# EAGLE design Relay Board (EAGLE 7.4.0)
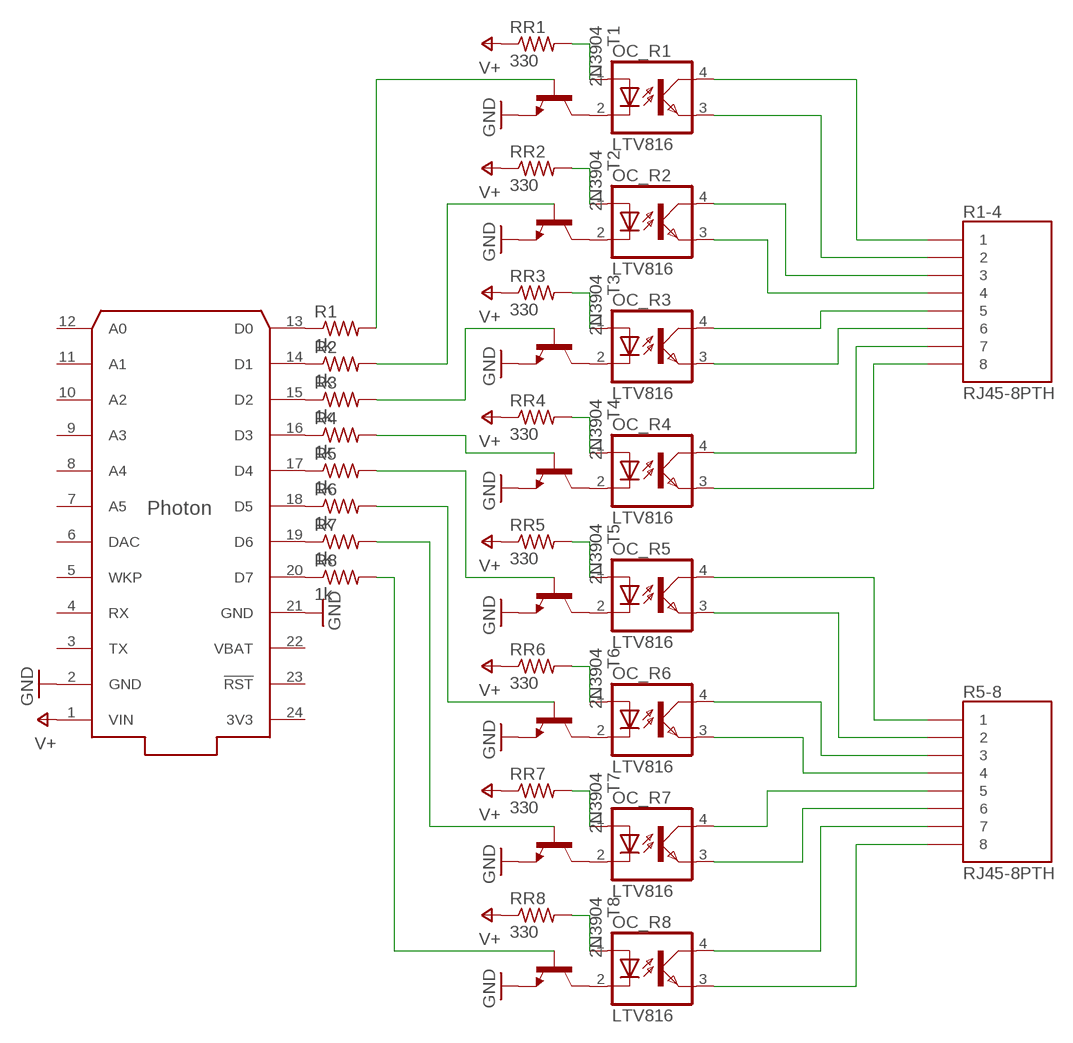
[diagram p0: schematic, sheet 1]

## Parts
OC_R1  LTV816  [DIL04]
OC_R2  LTV816  [DIL04]
OC_R3  LTV816  [DIL04]
OC_R4  LTV816  [DIL04]
OC_R5  LTV816  [DIL04]
OC_R6  LTV816  [DIL04]
OC_R7  LTV816  [DIL04]
OC_R8  LTV816  [DIL04]
PHOTON  PHOTON_WITH_HEADERS  [PHOTON]
R1  1k  R-US_0204/7  [0204/7]
R1-4  RJ45-8PTH  [RJ45-8]
R2  1k  R-US_0204/7  [0204/7]
R3  1k  R-US_0204/7  [0204/7]
R4  1k  R-US_0204/7  [0204/7]
R5  1k  R-US_0204/7  [0204/7]
R5-8  RJ45-8PTH  [RJ45-8]
R6  1k  R-US_0204/7  [0204/7]
R7  1k  R-US_0204/7  [0204/7]
R8  1k  R-US_0204/7  [0204/7]
RR1  330  R-US_0204/7  [0204/7]
RR2  330  R-US_0204/7  [0204/7]
RR3  330  R-US_0204/7  [0204/7]
RR4  330  R-US_0204/7  [0204/7]
RR5  330  R-US_0204/7  [0204/7]
RR6  330  R-US_0204/7  [0204/7]
RR7  330  R-US_0204/7  [0204/7]
RR8  330  R-US_0204/7  [0204/7]
T1  2N3904  [TO92]
T2  2N3904  [TO92]
T3  2N3904  [TO92]
T4  2N3904  [TO92]
T5  2N3904  [TO92]
T6  2N3904  [TO92]
T7  2N3904  [TO92]
T8  2N3904  [TO92]

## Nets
GND: PHOTON.2(GND) PHOTON.21(GND) T1.3(E) T2.3(E) T3.3(E) T4.3(E) T5.3(E) T6.3(E) T7.3(E) T8.3(E)
N$1: PHOTON.13(D0) R1.1
N$2: PHOTON.14(D1) R2.1
N$3: PHOTON.15(D2) R3.1
N$4: PHOTON.16(D3) R4.1
N$5: PHOTON.17(D4) R5.1
N$6: PHOTON.18(D5) R6.1
N$7: PHOTON.19(D6) R7.1
N$8: PHOTON.20(D7) R8.1
N$9: OC_R1.4(COL) R1-4.1
N$10: OC_R1.3(EMIT) R1-4.2
N$11: OC_R2.4(COL) R1-4.3
N$12: OC_R2.3(EMIT) R1-4.4
N$13: OC_R3.4(COL) R1-4.5
N$14: OC_R3.3(EMIT) R1-4.6
N$15: OC_R4.4(COL) R1-4.7
N$16: OC_R4.3(EMIT) R1-4.8
N$17: OC_R5.4(COL) R5-8.1
N$18: OC_R5.3(EMIT) R5-8.2
N$19: OC_R6.4(COL) R5-8.3
N$20: OC_R6.3(EMIT) R5-8.4
N$21: OC_R7.4(COL) R5-8.5
N$22: OC_R7.3(EMIT) R5-8.6
N$23: OC_R8.4(COL) R5-8.7
N$24: OC_R8.3(EMIT) R5-8.8
N$25: OC_R8.2(C) T8.1(C)
N$26: OC_R7.2(C) T7.1(C)
N$27: OC_R6.2(C) T6.1(C)
N$28: OC_R5.2(C) T5.1(C)
N$29: OC_R4.2(C) T4.1(C)
N$30: OC_R3.2(C) T3.1(C)
N$31: OC_R2.2(C) T2.1(C)
N$32: OC_R1.2(C) T1.1(C)
N$33: OC_R1.1(A) RR1.2
N$34: OC_R2.1(A) RR2.2
N$35: OC_R3.1(A) RR3.2
N$36: OC_R4.1(A) RR4.2
N$37: OC_R5.1(A) RR5.2
N$38: OC_R6.1(A) RR6.2
N$39: OC_R7.1(A) RR7.2
N$40: OC_R8.1(A) RR8.2
N$41: R1.2 T1.2(B)
N$42: R2.2 T2.2(B)
N$43: R3.2 T3.2(B)
N$44: R4.2 T4.2(B)
N$45: R5.2 T5.2(B)
N$46: R6.2 T6.2(B)
N$47: R7.2 T7.2(B)
N$48: R8.2 T8.2(B)
V+: PHOTON.1(VIN) RR1.1 RR2.1 RR3.1 RR4.1 RR5.1 RR6.1 RR7.1 RR8.1
Unconnected: PHOTON.3(TX) PHOTON.4(RX) PHOTON.5(WKP) PHOTON.6(DAC) PHOTON.7(A5) PHOTON.8(A4) PHOTON.9(A3) PHOTON.10(A2) PHOTON.11(A1) PHOTON.12(A0) PHOTON.23(!RST)

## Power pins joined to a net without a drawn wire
3V3: PHOTON.24(3V3)
VBAT: PHOTON.22(VBAT)

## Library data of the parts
OC_R1-OC_R8 = optocoupler:LTV816: OPTO COUPLER Source: LITEON, LTV816.pdf; OC_FARNELL: unknown; OC_NEWARK: unknown
PHOTON = Spark:PHOTON
R1-R8 RR1-RR8 = rcl:R-US_: RESISTOR, American symbol
R1-4 R5-8 = SparkFun-Connectors:RJ45-8: RJ45 Jack Simple RJ45, 8-pin connection - connector for common Cat5, Cat5e, and Cat6 Ethernet cables. Footprint not yet proven in production. Connector sku is PRT-00643; Breakout PCB sku is BOB-00716.
T1-T8 = transistor:2N3904: NPN TRANSISTOR

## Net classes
0 default: width 0.305 mm, drill 0.508 mm, clearance 0.254 mm

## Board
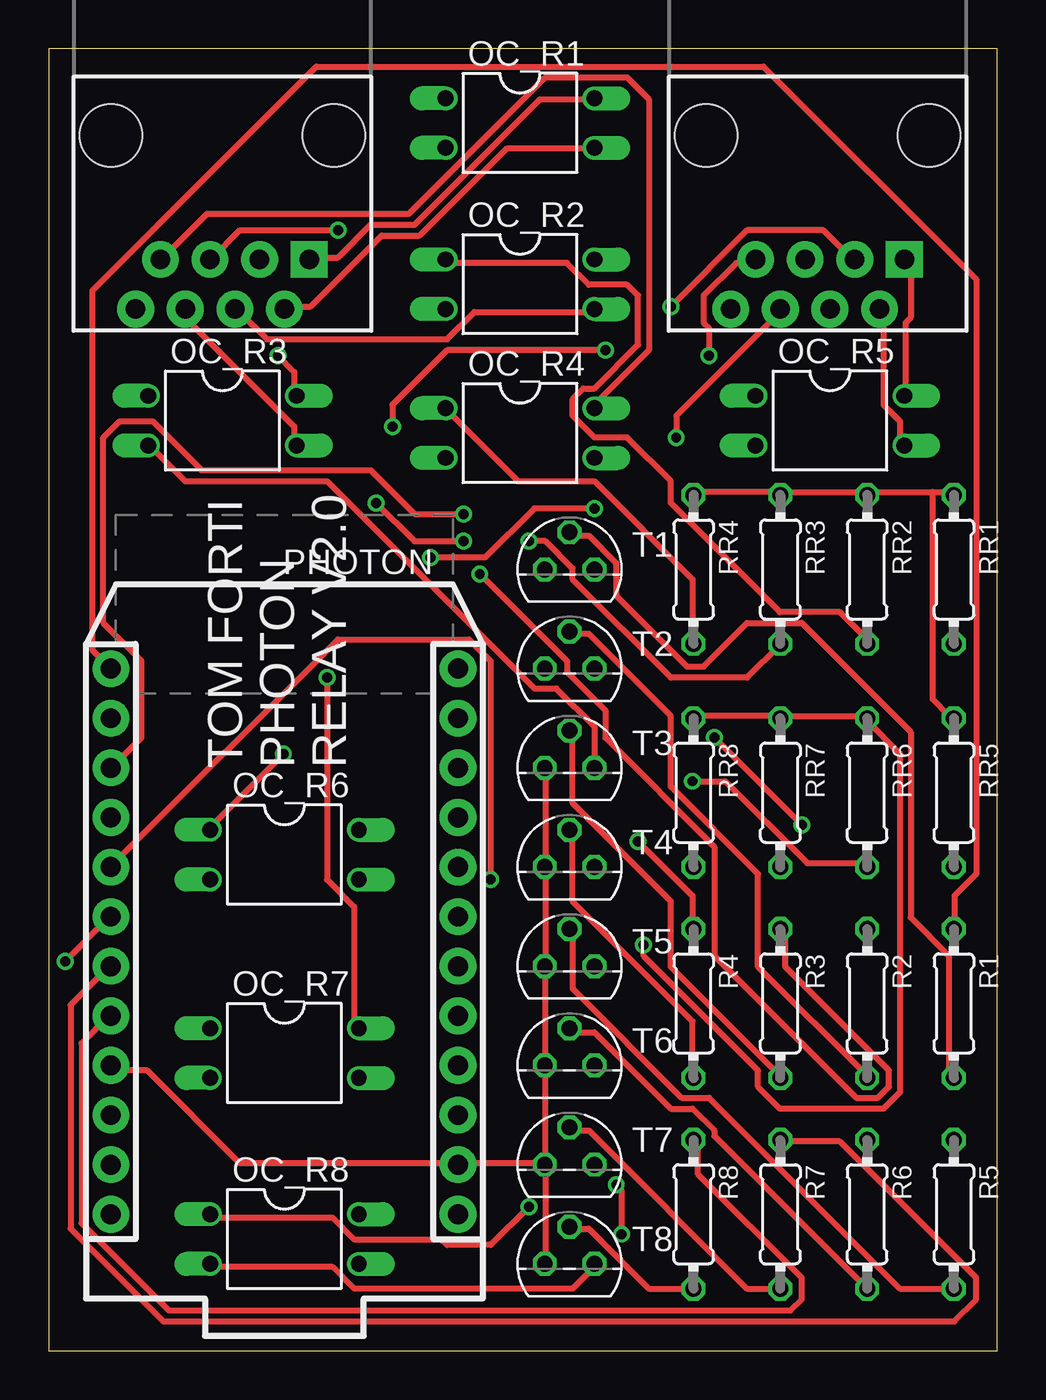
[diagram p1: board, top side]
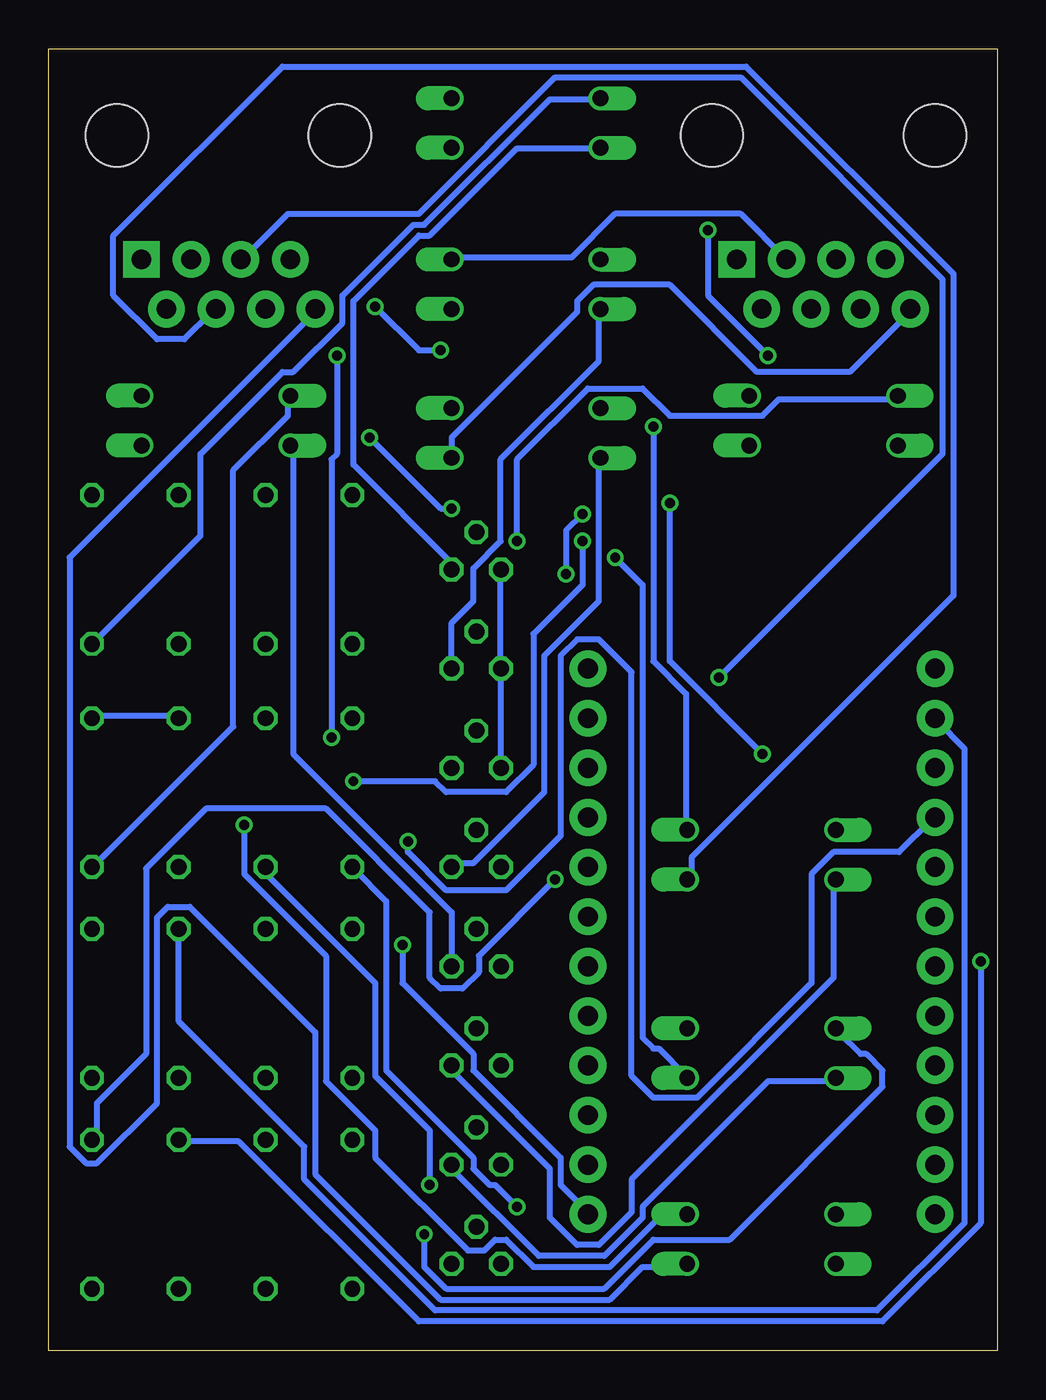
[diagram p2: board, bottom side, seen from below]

Size 48.56 x 66.67 mm. Coordinates in mm from the lower left corner, seen from the top.
Outline: 0,0 48.56,0 48.56,66.67 0,66.67 0,0
Copper layers (1*16): Top 0.0356mm / dielectric 1.5011mm / Bottom 0.0356mm
Design rules "LaenPCBOrder": minimum track width 6mil, minimum drill 13mil, track to track 6mil, track to pad 6mil, pad to pad 6mil, via to via 6mil, smd to smd 6mil, copper to edge 15mil, drill to drill 6mil, minimum pad ring 7mil, minimum via ring 7mil, stop-mask expansion 3mil, vias tented up to drill 0mil, thermal gap 10mil

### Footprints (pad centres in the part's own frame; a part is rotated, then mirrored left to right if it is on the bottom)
DIL04 = drill 0.813 offset: 1 -1.27,-3.81; 2 1.27,-3.81; 3 1.27,3.81; 4 -1.27,3.81
PHOTON = drill 1.016 pad 1.88: 1 1.27,32.258; 2 1.27,29.718; 3 1.27,27.178; 4 1.27,24.638; 5 1.27,22.098; 6 1.27,19.558; 7 1.27,17.018; 8 1.27,14.478; 9 1.27,11.938; 10 1.27,9.398; 11 1.27,6.858; 12 1.27,4.318; 13 19.05,4.318; 14 19.05,6.858; 15 19.05,9.398; 16 19.05,11.938; 17 19.05,14.478; 18 19.05,17.018; 19 19.05,19.558; 20 19.05,22.098; 21 19.05,24.638; 22 19.05,27.178; 23 19.05,29.718; 24 19.05,32.258
0204/7 = drill 0.813 octagon: 1 -3.81,0; 2 3.81,0
RJ45-8 = drill 1 pad 1.88 square: 1 -4.445,6.35 | drill 1 pad 1.88: 2 -3.175,8.89; 3 -1.905,6.35; 4 -0.635,8.89; 5 0.635,6.35; 6 1.905,8.89; 7 3.175,6.35; 8 4.445,8.89 | hole 3.2: -5.715,0; 5.715,0
TO92 = drill 0.813 octagon: 1 1.27,0; 2 0,1.905; 3 -1.27,0

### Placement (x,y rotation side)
OC_R1  24.13,62.86 270 top
OC_R2  24.13,54.61 270 top
OC_R3  8.89,47.62 270 top
OC_R4  24.13,46.99 270 top
OC_R5  40.01,47.62 270 top
OC_R6  12.06,25.4 270 top
OC_R7  12.06,15.24 270 top
OC_R8  12.06,5.71 270 top
PHOTON  22.23,39.24 180 top
R1  46.35,17.78 270 top
R1-4  8.89,62.23 180 top
R2  41.91,17.78 270 top
R3  37.47,17.78 270 top
R4  33.02,17.78 270 top
R5  46.35,6.98 270 top
R5-8  39.37,62.23 180 top
R6  41.91,6.98 270 top
R7  37.47,6.98 270 top
R8  33.02,6.98 270 top
RR1  46.35,40 270 top
RR2  41.91,40 270 top
RR3  37.47,40 270 top
RR4  33.02,40 270 top
RR5  46.35,28.57 270 top
RR6  41.91,28.57 270 top
RR7  37.47,28.57 270 top
RR8  33.02,28.57 270 top
T1  26.67,40 0 top
T2  26.67,34.92 0 top
T3  26.67,29.85 0 top
T4  26.67,24.77 0 top
T5  26.67,19.69 0 top
T6  26.67,14.61 0 top
T7  26.67,9.52 0 top
T8  26.67,4.45 0 top

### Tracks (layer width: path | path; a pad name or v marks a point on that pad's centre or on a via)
GND
  Top 0.305: T3.3 25.43,29.72 25.43,24.97 T4.3 25.43,24.69 25.43,19.94 T5.3 25.43,19.66 25.43,14.63 T6.3 25.43,14.35 25.43,9.6 T7.3 | T8.3 25.43,4.57 25.43,9.32 T7.3 | 20.95,9.6 25.15,9.6 T7.3 | 20.95,9.6 9.78,9.6 5.03,14.35 3.35,14.35 PHOTON.21 | 20.95,9.6 PHOTON.2
  Bottom 0.305: T3.3 25.43,30 25.43,34.75 T2.3 25.43,35.03 25.43,39.78 T1.3
N$1
  Top 0.305: PHOTON.13 2.23,35.86 2.23,54.3 13.69,65.76 36.6,65.76 47.5,54.86 47.5,24.41 46.38,23.29 46.38,21.62 R1.1
N$2
  Bottom 0.305: R2.1 41.91,16.87 35.48,10.44 35.48,8.76 28.78,2.06 6.15,2.06 1.68,6.53 1.68,30.84 3.07,32.23 PHOTON.14
N$3  (via drill 0.51)
  Top 0.305: v22.07,39.78 26.54,35.31 26.54,34.75 28.5,32.79 28.5,31.39 34.09,25.81 34.09,20.22 41.35,12.95 42.47,12.95 43.03,13.51 43.03,14.35 37.72,19.66 37.72,21.34 R3.1 | v21.23,42.85 18.72,42.85 16.48,45.08 7.82,45.08 5.31,47.6 3.63,47.6 2.79,46.76 2.79,37.26 4.75,35.31 4.75,31.39 3.35,30 PHOTON.15
  Bottom 0.305: v22.07,39.78 22.07,42.01 v21.23,42.85
N$4  (via drill 0.51)
  Top 0.305: v30.18,26.09 32.97,23.29 32.97,21.62 R4.1
  Bottom 0.305: v30.18,26.09 30.18,25.53 28.22,23.57 25.15,23.57 22.35,26.37 22.35,35.58 21.51,36.42 20.4,36.42 18.72,34.75 18.72,14.07 17.6,12.95 15.37,12.95 9.5,18.82 9.5,24.41 8.38,25.53 5.03,25.53 3.35,27.2 PHOTON.16
N$5  (via drill 0.51)
  Top 0.305: v22.63,24.13 22.63,35.31 21.51,36.42 14.81,36.42 3.35,24.97 PHOTON.17
  Bottom 0.305: v22.63,24.13 26.54,20.22 26.54,19.38 27.38,18.54 28.5,18.54 29.06,19.1 29.06,22.45 34.37,27.76 40.51,27.76 43.59,24.69 43.59,15.19 46.1,12.68 46.1,11 R5.1
N$6  (via drill 0.51)
  Top 0.305: v0.84,19.94 3.07,22.17 PHOTON.18
  Bottom 0.305: v0.84,19.94 0.84,6.53 5.87,1.5 29.62,1.5 38.84,10.72 41.91,10.72 R6.1
N$7
  Top 0.305: R7.1 37.72,10.72 40.51,10.72 47.5,3.73 47.5,2.62 46.38,1.5 5.87,1.5 1.12,6.25 1.12,17.7 3.07,19.66 PHOTON.19
N$8
  Top 0.305: R8.1 33.25,10.72 33.25,9.04 38.56,3.73 38.56,2.62 38,2.06 6.15,2.06 1.68,6.53 1.68,15.75 3.07,17.14 PHOTON.20
N$9
  Top 0.305: OC_R1.4 27.94,64.08 25.15,64.08 18.72,57.66 16.48,57.66 14.81,55.98 13.41,55.98 R1-4.1
N$10
  Top 0.305: OC_R1.3 27.94,61.57 23.47,61.57 19,57.1 17.04,57.1 13.41,53.47 12.29,53.47 R1-4.2
N$11
  Bottom 0.305: R1-4.3 13.13,58.22 19.56,58.22 21.79,55.98 27.94,55.98 OC_R2.4
N$12
  Top 0.305: OC_R2.3 27.94,53.19 21.79,53.19 20.4,51.79 11.18,51.79 9.78,53.19 R1-4.4
N$13  (via drill 0.51)
  Top 0.305: v11.73,50.95 12.57,50.11 12.57,49 OC_R3.4 | v14.81,57.38 9.78,57.38 8.38,55.98 R1-4.5
  Bottom 0.305: v11.73,50.95 14.81,54.03 v14.81,57.38
N$14
  Top 0.305: R1-4.6 6.99,52.91 12.57,47.32 12.57,46.48 OC_R3.3
N$15
  Top 0.305: OC_R4.4 27.94,48.44 30.73,51.23 30.73,64.08 29.62,65.2 25.43,65.2 18.44,58.22 8.1,58.22 5.87,55.98 R1-4.7
N$16
  Bottom 0.305: OC_R4.3 27.94,46.76 21.51,53.19 21.51,53.75 20.68,54.58 16.76,54.58 12.29,50.11 7.54,50.11 4.47,53.19 R1-4.8
N$17
  Top 0.305: OC_R5.4 43.87,49 43.87,52.63 44.15,52.91 44.15,55.42 43.87,55.7 R5-8.1
N$18
  Top 0.305: OC_R5.3 43.59,46.48 43.59,47.6 42.75,48.44 42.75,53.19 R5-8.2
N$19  (via drill 0.51)
  Top 0.305: v17.6,47.32 17.6,48.44 20.4,51.23 v28.5,51.23 | v31.85,53.47 35.76,57.38 39.67,57.38 41.07,55.98 R5-8.3
  Bottom 0.305: v17.6,47.32 17.6,35.31 15.93,33.63 15.93,26.92 OC_R6.4 | v28.5,51.23 29.62,51.23 v31.85,53.47
N$20
  Bottom 0.305: OC_R6.3 15.65,24.13 15.65,25.25 2.23,38.66 2.23,55.14 12.85,65.76 36.6,65.76 45.26,57.1 45.26,54.03 43.03,51.79 41.63,51.79 40.23,53.19 R5-8.4
N$21  (via drill 0.51)
  Top 0.305: v14.25,34.47 14.25,24.13 15.65,22.73 15.65,16.59 OC_R7.4
  Bottom 0.305: v14.25,34.47 2.79,45.92 2.79,54.86 13.13,65.2 22.63,65.2 29.62,58.22 36.32,58.22 38.56,55.98 R5-8.5
N$22  (via drill 0.51)
  Top 0.305: v19.56,40.61 22.35,40.61 24.87,43.13 v27.94,43.13 | v32.13,46.76 32.13,47.88 37.44,53.19 R5-8.6
  Bottom 0.305: v19.56,40.61 18.16,39.22 18.16,16.03 17.6,15.47 17.32,15.47 15.93,14.07 OC_R7.3 | v27.94,43.13 28.5,43.13 v32.13,46.76
N$23  (via drill 0.51)
  Top 0.305: v34.09,31.39 v38.56,26.92 | v33.81,50.95 33.81,52.35 33.53,52.63 33.53,54.03 35.2,55.7 36.04,55.7 R5-8.7
  Bottom 0.305: v38.56,26.92 38.56,24.41 34.37,20.22 34.37,13.79 31.85,11.28 31.85,9.88 27.1,5.13 26.26,5.13 25.7,5.69 25.15,5.69 23.75,4.29 19.84,4.29 17.32,6.81 15.93,6.81 OC_R8.4 | v34.09,31.39 34.09,45.64 33.81,45.92 v33.81,50.95
N$24
  Bottom 0.305: OC_R8.3 15.93,4.29 18.16,4.29 19.84,2.62 28.5,2.62 34.92,9.04 34.92,16.31 41.35,22.73 42.47,22.73 43.03,22.17 43.03,12.68 46.1,9.6 46.66,9.6 47.5,10.44 47.5,40.61 34.92,53.19 R5-8.8
N$25
  Top 0.305: OC_R8.2 8.38,4.29 14.53,4.29 15.65,3.17 26.82,3.17 27.94,4.29 T8.1
N$26
  Bottom 0.305: T7.1 27.94,9.32 23.47,4.85 20.12,4.85 18.16,6.81 18.16,7.37 11.73,13.79 8.38,13.79 OC_R7.2
N$27
  Bottom 0.305: T6.1 27.94,14.35 22.91,9.32 22.91,6.81 21.51,5.41 20.4,5.41 18.72,7.09 18.72,8.76 8.38,19.1 8.38,24.13 OC_R6.2
N$28
  Bottom 0.305: T5.1 27.94,22.45 36.04,30.56 36.04,46.2 OC_R5.2
N$29
  Bottom 0.305: OC_R4.2 20.4,45.64 20.4,38.38 23.19,35.58 23.19,28.6 26.82,24.97 27.94,24.97 T4.1
N$30
  Top 0.305: T3.1 27.94,31.95 25.98,33.91 24.87,33.91 14.25,44.53 6.99,44.53 5.31,46.2 OC_R3.2
N$31
  Bottom 0.305: T2.1 27.94,37.26 26.82,38.38 26.82,40.06 25.43,41.45 25.43,45.64 20.4,50.67 20.4,53.19 OC_R2.2
N$32
  Bottom 0.305: T1.1 27.94,40.33 32.97,45.36 32.97,53.75 29.62,57.1 29.06,57.1 24.59,61.57 20.4,61.57 OC_R1.2
N$33
  Bottom 0.305: OC_R1.1 20.4,64.08 22.91,64.08 29.34,57.66 29.9,57.66 33.53,54.03 33.53,52.63 36.04,50.11 36.6,50.11 40.79,45.92 40.79,41.73 46.1,36.42 RR1.2
N$34
  Top 0.305: OC_R2.1 20.4,55.7 26.54,55.7 27.66,54.58 29.62,54.58 30.18,54.03 30.18,51.51 27.94,49.28 27.38,49.28 26.82,48.72 26.82,47.88 27.94,46.76 29.62,46.76 31.85,44.53 31.85,43.41 37.44,37.82 40.51,37.82 41.91,36.42 RR2.2
N$35  (via drill 0.51)
  Top 0.305: v24.59,41.45 25.43,41.45 26.82,40.06 26.82,39.5 31.85,34.47 35.76,34.47 37.44,36.14 RR3.2
  Bottom 0.305: v24.59,41.45 24.59,45.64 20.95,49.28 18.16,49.28 16.76,47.88 12.01,47.88 11.18,48.72 5.31,48.72 OC_R3.1
N$36
  Top 0.305: RR4.2 32.97,36.42 32.97,39.5 27.94,44.53 24.03,44.53 20.4,48.16 OC_R4.1
N$37
  Bottom 0.305: OC_R5.1 36.32,48.72 36.32,47.88 39.12,45.08 39.12,31.95 46.1,24.97 RR5.2
N$38  (via drill 0.51)
  Top 0.305: v32.97,29.16 34.65,29.16 38.84,24.97 41.91,24.97 RR6.2 | v21.23,41.45 18.72,41.45 v16.76,43.41 | v12.01,30.56 8.38,26.92 OC_R6.1
  Bottom 0.305: v32.97,29.16 28.78,29.16 28.22,28.6 25.15,28.6 23.75,30 23.75,36.7 21.23,39.22 v21.23,41.45 | v16.76,43.41 16.76,35.31 v12.01,30.56
N$39  (via drill 0.51)
  Top 0.305: v29.34,5.97 29.34,8.2 v29.06,8.48
  Bottom 0.305: v29.34,5.97 29.34,4.29 28.22,3.17 20.12,3.17 17.6,5.69 13.69,5.69 5.87,13.51 5.87,14.35 6.71,15.19 6.99,15.19 8.1,16.31 OC_R7.1 | v29.06,8.48 29.06,11.28 31.85,14.07 31.85,18.82 37.72,24.69 RR7.2
N$40  (via drill 0.51)
  Top 0.305: v24.59,7.37 22.63,5.41 20.4,5.41 20.12,5.69 15.65,5.69 14.53,6.81 8.38,6.81 OC_R8.1
  Bottom 0.305: v24.59,7.37 25.7,8.48 25.98,8.48 26.82,9.32 26.82,9.88 31.29,14.35 31.29,23.01 32.97,24.69 RR8.2
N$41
  Top 0.305: R1.2 46.1,14.07 46.1,20.22 44.15,22.17 44.15,31.67 38.56,37.26 35.76,37.26 33.53,35.03 32.69,35.03 29.06,38.66 29.06,40.33 27.66,41.73 26.82,41.73 T1.2
N$42
  Top 0.305: T2.2 26.82,36.7 27.66,36.7 31.85,32.51 31.85,28.88 36.32,24.41 36.32,19.66 41.91,14.07 R2.2
N$43
  Top 0.305: T3.2 26.82,31.67 26.82,28.04 31.85,23.01 31.85,19.66 37.44,14.07 R3.2
N$44
  Top 0.305: T4.2 26.82,26.64 26.82,23.01 32.97,16.87 32.97,14.07 R4.2
N$45
  Top 0.305: R5.2 43.59,3.17 33.81,12.95 32.41,12.95 26.82,18.54 26.82,21.34 T5.2
N$46
  Top 0.305: R6.2 34.09,11 34.09,11.28 32.97,12.39 31.85,12.39 27.94,16.31 26.82,16.31 T6.2
N$47
  Top 0.305: R7.2 35.76,3.17 27.66,11.28 26.82,11.28 T7.2
N$48
  Top 0.305: R8.2 30.73,3.17 27.66,6.25 26.82,6.25 T8.2
V+  (via drill 0.51)
  Top 0.305: RR4.1 33.25,43.97 37.44,43.97 RR3.1 37.72,43.97 41.91,43.97 | 41.91,43.97 45.26,43.97 | 45.26,43.97 46.1,43.97 RR1.1 | 41.91,43.97 RR2.1 | RR8.1 33.25,32.51 37.44,32.51 RR7.1 37.72,32.51 41.91,32.51 RR6.1 41.91,32.23 43.59,30.56 43.59,13.23 42.75,12.39 37.44,12.39 36.32,13.51 36.32,14.35 30.45,20.22 v30.45,20.78 | 45.26,43.97 45.26,33.35 46.1,32.51 RR5.1
  Bottom 0.305: RR5.1 46.1,32.51 41.91,32.51 RR6.1 | v30.45,20.78 30.45,18.82 26.82,15.19 26.82,14.35 22.35,9.88 22.35,8.48 20.95,7.09 PHOTON.1

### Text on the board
tPlace: TOM FORTI / PHOTON / RELAY V2.0

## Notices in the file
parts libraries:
SparkFun-Connectors: Licensing: CC v3.0 Share-Alike You are welcome to use this library for commercial purposes.
